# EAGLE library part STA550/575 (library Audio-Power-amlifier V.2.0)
STA575 100+100W STEREO POWER AMPLIFIER STA550 70+70W STEREO POWER AMPLIFIER
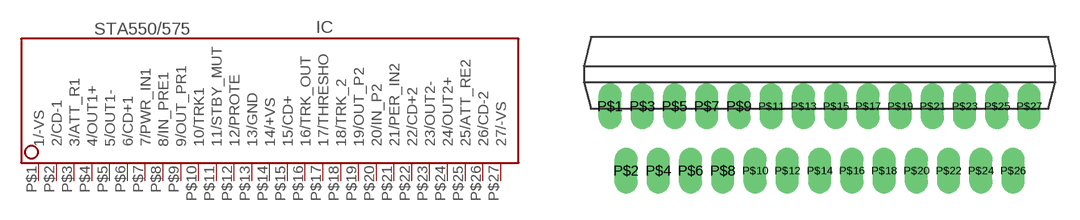
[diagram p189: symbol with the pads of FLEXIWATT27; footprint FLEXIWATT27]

Designator prefix IC

## STA550/575  [FLEXIWATT27]
P$1  1/-VS  pwr
P$2  2/CD-1  pwr
P$3  3/ATT_R1
P$4  4/OUT1+  out
P$5  5/OUT1-  out
P$6  6/CD+1  pwr
P$7  7/PWR_IN1  in
P$8  8/IN_PRE1  in
P$9  9/OUT_PR1  out
P$10  10/TRK1  in
P$11  11/STBY_MUT  in
P$12  12/PROTE
P$13  13/GND  pwr
P$14  14/+VS  pwr
P$15  15/CD+  pwr
P$16  16/TRK_OUT  out
P$17  17/THRESHO  in
P$18  18/TRK_2  in
P$19  19/OUT_P2  out
P$20  20/IN_P2  in
P$21  21/PER_IN2  in
P$22  22/CD+2  pwr
P$23  23/OUT2-  out
P$24  24/OUT2+  out
P$25  25/ATT_RE2
P$26  26/CD-2  pwr
P$27  27/-VS  pwr

## Footprint FLEXIWATT27 (pad centres in mm)
Flexiwatt27
drill 0.7 pad 1.422 long: P$1 -13,0; P$2 -12,-4; P$3 -11,0; P$4 -10,-4; P$5 -9,0; P$6 -8,-4; P$7 -7,0; P$8 -6,-4; P$9 -5,0; P$10 -4,-4; P$11 -3,0; P$12 -2,-4; P$13 -1,0; P$14 0,-4; P$15 1,0; P$16 2,-4; P$17 3,0; P$18 4,-4; P$19 5,0; P$20 6,-4; P$21 7,0; P$22 8,-4; P$23 9,0; P$24 10,-4; P$25 11,0; P$26 12,-4; P$27 13,0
